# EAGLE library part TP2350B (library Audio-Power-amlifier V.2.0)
The TP2350B is a two-channel, 300W (4Ω) per channel Amplifier Driver that uses Tripath’s proprietary Digital Power Processing (DPPTM) technology. Class-T amplifiers offer both the audio fidelity of Class-AB and the power efficiency of Class-D amplifiers.
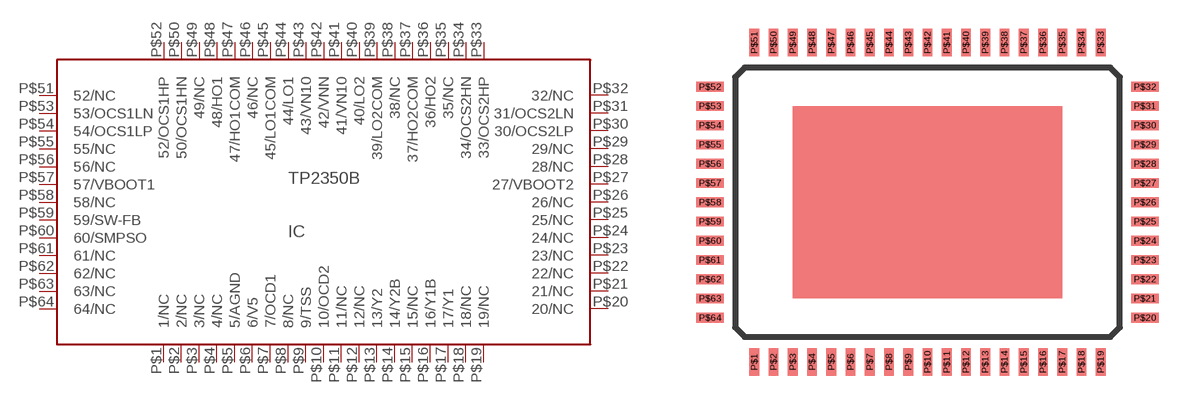
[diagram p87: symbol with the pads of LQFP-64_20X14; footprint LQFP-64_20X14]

Designator prefix IC

## TP2350B  [LQFP-64_20X14]
P$1  1/NC  nc
P$2  2/NC  nc
P$3  3/NC  nc
P$4  4/NC  nc
P$5  5/AGND  pwr
P$6  6/V5  pwr
P$7  7/OCD1
P$8  8/NC  nc
P$9  9/TSS
P$10  10/OCD2
P$11  11/NC  nc
P$12  12/NC  nc
P$13  13/Y2
P$14  14/Y2B
P$15  15/NC  nc
P$16  16/Y1B
P$17  17/Y1
P$18  18/NC  nc
P$19  19/NC  nc
P$20  20/NC  nc
P$21  21/NC  nc
P$22  22/NC  nc
P$23  23/NC  nc
P$24  24/NC  nc
P$25  25/NC  nc
P$26  26/NC  nc
P$27  27/VBOOT2
P$28  28/NC  nc
P$29  29/NC  nc
P$30  30/OCS2LP
P$31  31/OCS2LN
P$32  32/NC  nc
P$33  33/OCS2HP
P$34  34/OCS2HN
P$35  35/NC  nc
P$36  36/HO2  out
P$37  37/HO2COM
P$38  38/NC  nc
P$39  39/LO2COM
P$40  40/LO2  out
P$41  41/VN10
P$42  42/VNN
P$43  43/VN10
P$44  44/LO1  out
P$45  45/LO1COM
P$46  46/NC  nc
P$47  47/HO1COM
P$48  48/HO1  out
P$49  49/NC  nc
P$50  50/OCS1HN
P$51  52/NC  nc
P$52  52/OCS1HP
P$53  53/OCS1LN
P$54  54/OCS1LP
P$55  55/NC  nc
P$56  56/NC  nc
P$57  57/VBOOT1
P$58  58/NC  nc
P$59  59/SW-FB
P$60  60/SMPSO
P$61  61/NC  nc
P$62  62/NC  nc
P$63  63/NC  nc
P$64  64/NC  nc

## Footprint LQFP-64_20X14 (pad centres in mm)
64-PIN-LQFP_20x14
smd 0.5 x 1.422: P$1 -9,-8.3; P$2 -8,-8.3; P$3 -7,-8.3; P$4 -6,-8.3; P$5 -5,-8.3; P$6 -4,-8.3; P$7 -3,-8.3; P$8 -2,-8.3; P$9 -1,-8.3; P$10 0,-8.3; P$11 1,-8.3; P$12 2,-8.3; P$13 3,-8.3; P$14 4,-8.3; P$15 5,-8.3; P$16 6,-8.3; P$17 7,-8.3; P$18 8,-8.3; P$19 9,-8.3; P$33 9,8.3; P$34 8,8.3; P$35 7,8.3; P$36 6,8.3; P$37 5,8.3; P$38 4,8.3; P$39 3,8.3; P$40 2,8.3; P$41 1,8.3; P$42 0,8.3; P$43 -1,8.3; P$44 -2,8.3; P$45 -3,8.3; P$46 -4,8.3; P$47 -5,8.3; P$48 -6,8.3; P$49 -7,8.3; P$50 -8,8.3; P$51 -9,8.3
smd 1.422 x 0.5: P$20 11.3,-6; P$21 11.3,-5; P$22 11.3,-4; P$23 11.3,-3; P$24 11.3,-2; P$25 11.3,-1; P$26 11.3,0; P$27 11.3,1; P$28 11.3,2; P$29 11.3,3; P$30 11.3,4; P$31 11.3,5; P$32 11.3,6; P$52 -11.3,6; P$53 -11.3,5; P$54 -11.3,4; P$55 -11.3,3; P$56 -11.3,2; P$57 -11.3,1; P$58 -11.3,0; P$59 -11.3,-1; P$60 -11.3,-2; P$61 -11.3,-3; P$62 -11.3,-4; P$63 -11.3,-5; P$64 -11.3,-6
